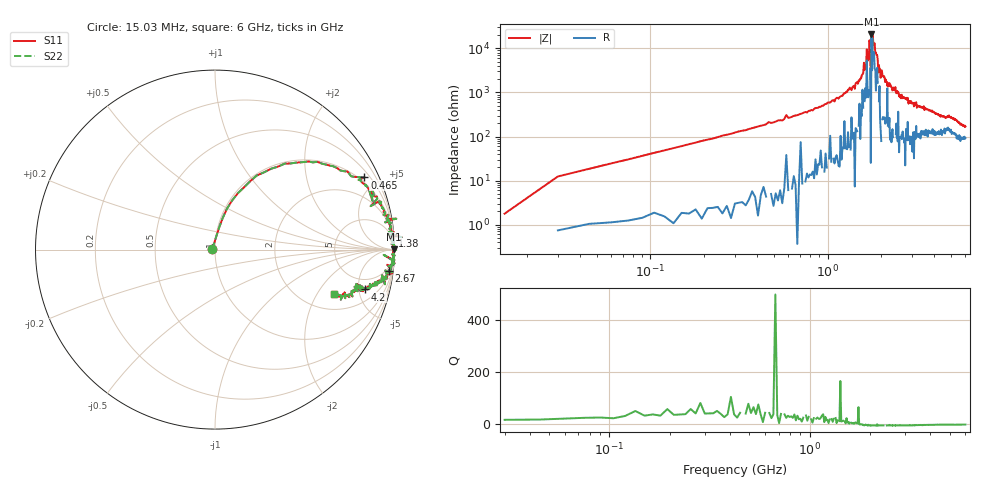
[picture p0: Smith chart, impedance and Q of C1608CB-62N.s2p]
!	Network	Analyzer	HP8753E.07.74:	Oct	30	2002	Serial	No.	JP38451487
!	Hewlett-Packard
!	28	Aug	2009	8:21:51
!	Frequency	S11	S21	S12	S22
#	HZ	S	RI	R	50
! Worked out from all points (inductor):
!   400 points, 15.03 MHz to 6 GHz, reference 50 ohm
!   read as one part in series: L = 64.8 nH near 45.03 MHz
!   highest |Z| = 20.8 kohm at 1.77 GHz (marker M1)
!   self-resonance near 1.77 GHz
!   S11 on the Smith chart (normalised r, x): 15.03 MHz: 0.97, +0.00; 465 MHz: 0.77, +4.24; 1.38 GHz: 3, +26; 2.67 GHz: 3, -16; 4.2 GHz: 3.29, -5.88; 6 GHz: 2.83, -2.86
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1.502992e7  -0.016 0.00103  1.02 -0.00103  1.02 -0.00103  -0.016 0.00103
3.002985e7  0.0221 0.12  0.978 -0.12  0.978 -0.12  0.0221 0.12
9.002955e7  0.127 0.314  0.873 -0.314  0.873 -0.314  0.127 0.314
4.650277e8  0.832 0.402  0.168 -0.402  0.168 -0.402  0.832 0.402
1.020025e9  0.964 0.162  0.0363 -0.162  0.0363 -0.162  0.964 0.162
1.380023e9  0.989 0.0754  0.011 -0.0754  0.011 -0.0754  0.989 0.0754
1.650022e9  0.994 0.0251  0.00574 -0.0251  0.00574 -0.0251  0.994 0.0251
1.665022e9  0.994 0.00861  0.00601 -0.00861  0.00601 -0.00861  0.994 0.00861
1.725021e9  1 0.0061  -0.00238 -0.0061  -0.00238 -0.0061  1 0.0061
1.740021e9  0.997 0.00897  0.00321 -0.00897  0.00321 -0.00897  0.997 0.00897
1.755021e9  0.995 0.0599  0.00452 -0.0599  0.00452 -0.0599  0.995 0.0599
1.770021e9  0.996 0.00235  0.00418 -0.00235  0.00418 -0.00235  0.996 0.00235
1.785021e9  0.992 -0.0131  0.0076 0.0131  0.0076 0.0131  0.992 -0.0131
1.800021e9  0.996 -0.00287  0.00388 0.00287  0.00388 0.00287  0.996 -0.00287
1.93502e9  0.999 -0.0352  0.000794 0.0352  0.000794 0.0352  0.999 -0.0352
2.01002e9  0.998 -0.0327  0.00192 0.0327  0.00192 0.0327  0.998 -0.0327
2.670017e9  0.97 -0.121  0.0299 0.121  0.0299 0.121  0.97 -0.121
3.015015e9  0.96 -0.161  0.0399 0.161  0.0399 0.161  0.96 -0.161
4.00501e9  0.864 -0.216  0.136 0.216  0.136 0.216  0.864 -0.216
4.200009e9  0.838 -0.222  0.162 0.222  0.162 0.222  0.838 -0.222
5.010005e9  0.79 -0.22  0.21 0.22  0.21 0.22  0.79 -0.22
6e9  0.665 -0.25  0.335 0.25  0.335 0.25  0.665 -0.25
